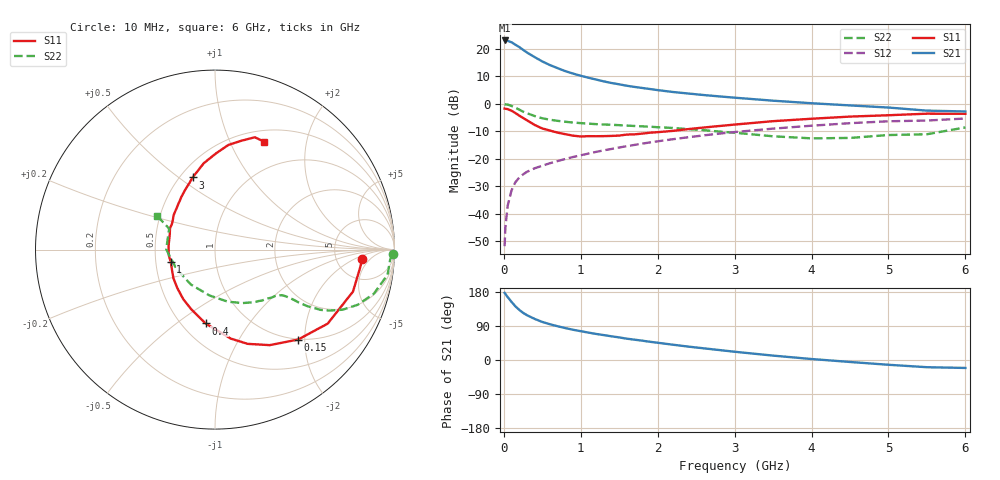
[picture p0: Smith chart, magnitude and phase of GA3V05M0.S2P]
! Infineon Technologies  Discrete & RF Semiconductors
! BF775
! Si NPN RF Bipolar Junction Transistor in SOT23
! VCE = 3 V  IC = 5 mA
! Common Emitter S-Parameters:  May  1996
# GHz  S  MA  R  50
!  f  S11  S21  S12  S22
! GHz  MAG  ANG  MAG  ANG  MAG  ANG  MAG  ANG
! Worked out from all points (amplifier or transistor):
!   36 points, 10 MHz to 6 GHz, reference 50 ohm
!   highest |S21| = 23.1 dB at 10 MHz (marker M1)
!   |S21| within 3 dB of that: start of sweep to 230.6 MHz
!   unconditionally stable (mu >= 1): 792 MHz to 3.506 GHz
!   at 250 MHz: K = 0.49, MSG = 22.6 dB, |S12| = -25.6 dB
!   at 1.4 GHz: K = 1.13, MAG = 9.8 dB, |S12| = -16.4 dB
!   at 6 GHz: K = 0.97, MSG = 1.3 dB, |S12| = -5.3 dB
!   lowest NFmin = 1.50 dB at 450 MHz
!   S11 on the Smith chart (normalised r, x): 10 MHz: 9.29, -2.86; 150 MHz: 0.99, -1.86; 400 MHz: 0.65, -0.64; 1 GHz: 0.60, -0.09; 3 GHz: 0.58, +0.56; 6 GHz: 0.63, +1.35
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0.01  0.821 -3.5  14.21 177.2  0.0026 91.2  0.9919 -1.5
0.02  0.8159 -6.6  13.96 174.2  0.0057 86.4  0.9777 -3.2
0.05  0.8037 -16.9  13.96 166.0  0.0142 81.5  0.9717 -8.3
0.1  0.7513 -33.3  13.16 153.4  0.0268 73.5  0.9186 -15.5
0.15  0.6821 -47.3  11.89 141.6  0.0378 66.8  0.8532 -21.1
0.2  0.6134 -60.2  10.8 132.3  0.0458 62.4  0.7866 -25.2
0.25  0.5557 -70.9  9.614 124.5  0.0523 59.0  0.7235 -28.0
0.3  0.5034 -80.0  8.584 118.3  0.0583 57.9  0.6779 -29.7
0.4  0.4146 -97.3  7.085 108.5  0.0675 55.6  0.6024 -31.5
0.5  0.3573 -111.9  5.904 100.4  0.0753 55.1  0.5477 -32.3
0.6  0.3277 -122.7  5.07 94.3  0.0836 55.2  0.5149 -32.6
0.8  0.2814 -145.3  3.934 84.2  0.1 55.9  0.4735 -33.4
1  0.2558 -164.6  3.243 76.0  0.1166 57.1  0.4472 -34.6
1.1  0.2593 -172.8  2.986 72.3  0.1252 57.1  0.4379 -35.8
1.3  0.2597 173.1  2.563 65.7  0.1433 56.9  0.4221 -37.9
1.6  0.2772 154.8  2.135 56.2  0.1707 55.8  0.4036 -42.2
2.2  0.3236 129.6  1.644 40.3  0.2283 52.2  0.365 -53.6
3  0.421 107.2  1.297 21.8  0.3078 44.3  0.2993 -76.0
3.5  0.4854 97.4  1.143 11.6  0.3553 38.4  0.2576 -96.8
4.5  0.5879 82.7  0.938 -5.2  0.4463 25.4  0.2408 -154.3
5.5  0.664 70.5  0.754 -19.0  0.4982 10.5  0.2808 155.4
6  0.6607 65.5  0.728 -21.0  0.5427 6.4  0.3738 149.8
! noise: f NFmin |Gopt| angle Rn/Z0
0.45  1.5  0.28  29  0.34
0.9  1.8  0.25  59  0.34
